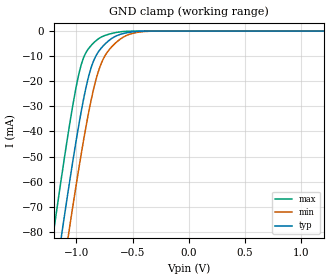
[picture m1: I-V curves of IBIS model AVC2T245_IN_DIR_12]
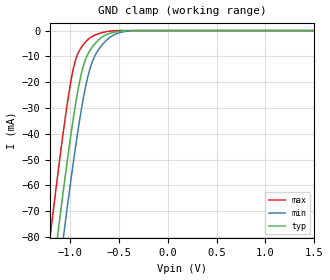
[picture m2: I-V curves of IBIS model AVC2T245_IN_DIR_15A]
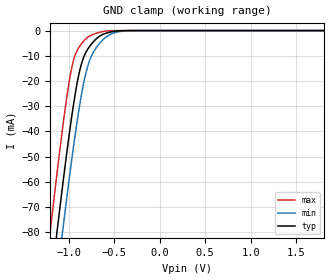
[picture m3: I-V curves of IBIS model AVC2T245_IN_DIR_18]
| TEXAS INSTRUMENTS INCORPORATED
| Standard Linear and Logic Group
| IBIS Model of SN74AVC2T245
| Dual-Bit Dual-Supply Bus Transceiver With Configurable Voltage
| Translation and 3-State Outputs
| This file contains package information for the following:
|  LGA 10-pin (RSW) package as [Component] SN74AVC2T245_RSW
| This device can be powered at the following Vccs:
|  1.2 volt Vcc
|  1.5 volt Vcc
|  1.8 volt Vcc
|  2.5 volt Vcc
|  3.3 volt Vcc
| This file provides unique models under the [Model Selector] for each Vcc.
| For operation at a specific Vcc, select the appropriate model after each
| [Model Selector] keyword.
[IBIS Ver]   3.2
[Comment char]  |_char
[File Name]   sn74avc2t245.ibs
[File Rev]   1.1 | x_die
[Date]   January 7, 2009
[Source]   Data created from TI-SPICE simulations at TI-SLL.
[Notes]   The following is an IBIS list for the SN74AVC2T245.
   Please contact sllibis@ti.com with questions and
   comments concerning SLL IBIS models.
   -FILE REV HISTORY
   -1.1 Release IBIS file on 01/08/09.
   -Power Clamp data deleted from control input model as there
   is no power-clamp diode.
[Disclaimer] Property of Texas Instruments Incorporated.  Unauthorized
   reproduction and/or distribution is strictly prohibited.
   This product is protected under copyright law.
   Created  2009, (C) Copyright  2009, Texas Instruments
   Incorporated, All Rights Reserved
   UNLESS THERE IS A SIGNED, WRITTEN AGREEMENT TO THE
   CONTRARY, TEXAS INSTRUMENTS (TI) IS PROVIDING THE IBIS
   MODELS  AND WITHOUT ANY WARRANTY, EXPRESSED OR
   IMPLIED.  TI assumes no liability for:
   1) the accuracy of the IBIS models provided to your
   company;
   2) the proper functioning of these IBIS Models in your
   design or for any resulting applications; or
   3) infringement of patents, copyrights or intellectual
   property rights resulting from your use of these IBIS
   models.
   TI provides IBIS Models as a service to our customers.
   You and your company shall not distribute, sell or give
   these models to anyone else without prior written
   permission from TI.
   TI reserves the right to make changes to our products or
   to discontinue any semiconductor product or service
   without notice, and advises our customers to obtain the
   latest version of relevant information to verify, before
   placing orders, that the information being relied on is
   current.
   Please be aware that your receipt and use of the IBIS
   information provided shall serve as acceptance of these
   terms and conditions.  If you do not accept these terms,
   you should return or destroy the IBIS models and any
   other accompanying information immediately.
| Component SN74AVC2T245_RSW 10-PIN LGA
[Component]   SN74AVC2T245_RSW
[Manufacturer]   Texas Instruments, Inc.
[Package]
|   typ   min   max
R_pkg   1.700e-02   1.500e-02   2.200e-02
L_pkg   5.570e-10   4.830e-10   6.520e-10
C_pkg   1.440e-13   1.050e-13   1.870e-13
[Pin]   signal_name   model_name   R_pin   L_pin   C_pin
1   DIR2   AVC2T245_IN_DIR   1.600e-02   4.830e-10   1.100e-13
2   NOE   AVC2T245_IN_NOE   1.500e-02   5.130e-10   1.860e-13
3   GND   GND   1.800e-02   5.860e-10   1.870e-13
4   B2   AVC2T245_IO   2.200e-02   6.520e-10   1.180e-13
5   B1   AVC2T245_IO   1.600e-02   5.500e-10   1.250e-13
6   VCCB   POWER   1.600e-02   4.830e-10   1.050e-13
7   VCCA   POWER   1.500e-02   5.150e-10   1.820e-13
8   A1   AVC2T245_IO   1.700e-02   5.790e-10   1.870e-13
9   A2   AVC2T245_IO   2.200e-02   6.360e-10   1.170e-13
10   DIR1   AVC2T245_IN_DIR   1.700e-02   5.710e-10   1.280e-13
| Model AVC2T245_IN_DIR
[Model Selector]   AVC2T245_IN_DIR
AVC2T245_IN_DIR_12   1.2 volt Vcc
AVC2T245_IN_DIR_15A   1.5 volt Vcc
AVC2T245_IN_DIR_18   1.8 volt Vcc
AVC2T245_IN_DIR_25   2.5 volt Vcc
AVC2T245_IN_DIR_33   3.3 volt Vcc
| Model AVC2T245_IN_NOE
[Model Selector]   AVC2T245_IN_NOE
AVC2T245_IN_NOE_12   1.2 volt Vcc
AVC2T245_IN_NOE_15A   1.5 volt Vcc
AVC2T245_IN_NOE_18   1.8 volt Vcc
AVC2T245_IN_NOE_25   2.5 volt Vcc
AVC2T245_IN_NOE_33   3.3 volt Vcc
| Model AVC2T245_IO
[Model Selector]   AVC2T245_IO
AVC2T245_IO_12   1.2 volt Vcc
AVC2T245_IO_15A   1.5 volt Vcc
AVC2T245_IO_18   1.8 volt Vcc
AVC2T245_IO_25   2.5 volt Vcc
AVC2T245_IO_33   3.3 volt Vcc
| Models and submodels in the file (15): AVC2T245_IN_DIR_12 (Input), AVC2T245_IN_DIR_15A (Input), AVC2T245_IN_DIR_18 (Input), AVC2T245_IN_DIR_25 (Input), AVC2T245_IN_DIR_33 (Input), AVC2T245_IN_NOE_12 (Input), AVC2T245_IN_NOE_15A (Input), AVC2T245_IN_NOE_18 (Input), AVC2T245_IN_NOE_25 (Input), AVC2T245_IN_NOE_33 (Input), AVC2T245_IO_12 (I/O), AVC2T245_IO_15A (I/O), AVC2T245_IO_18 (I/O), AVC2T245_IO_25 (I/O), AVC2T245_IO_33 (I/O)
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[Model]   AVC2T245_IN_DIR_12
Model_type  Input
Vinl=0.385
Vinh=0.845
| variable   typ   min   max
C_comp   2.12pF   1.85pF   2.57pF
[Temperature Range]   40   100   -40
| Ambient temperature   25   85   -40
[Voltage range]   1.2   1.1   1.3
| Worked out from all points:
|   GND clamp passes 1 mA (typ) near -0.58 V on its own axis
[GND Clamp]
| AVC2T245_IN_DIR_12
|   Voltage   I(typ)   I(min)   I(max)
-4.6V     -1.266A    -1.277A    -1.254A
-1.22V    -108.9mA   -127.3mA   -85.71mA
-1.195V   -101.1mA   -119.4mA   -77.82mA
-1.13V    -81mA      -99.35mA   -57.75mA
-1.065V   -61.6mA    -79.78mA   -38.73mA
-960mV    -32.94mA   -49.96mA   -14.03mA
-905mV    -20.72mA   -35.89mA   -7.898mA
-860mV    -13.49mA   -25.81mA   -5.335mA
-760mV    -5.854mA   -11.09mA   -2.009mA
-615mV    -1.4mA     -3.395mA   -339.9uA
-340mV    -6.933uA   -59.17uA   -50.62nA
1.2V      105.6pA    10.37nA    15.63pA
[Model]   AVC2T245_IN_DIR_15A
Model_type  Input
Vinl=0.49
Vinh=1.04
| variable   typ   min   max
C_comp   2.08pF   1.77pF   2.54pF
[Temperature Range]   40   100   -40
| Ambient temperature   25   85   -40
[Voltage range]   1.5   1.4   1.6
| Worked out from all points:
|   GND clamp passes 1 mA (typ) near -0.58 V on its own axis
[GND Clamp]
| AVC2T245_IN_DIR_15A
|   Voltage   I(typ)   I(min)   I(max)
-4.6V     -1.266A    -1.277A    -1.254A
-1.21V    -105.8mA   -124.1mA   -82.55mA
-1.185V   -97.95mA   -116.3mA   -74.69mA
-1.125V   -79.48mA   -97.82mA   -56.25mA
-1.06V    -60.14mA   -78.3mA    -37.34mA
-960mV    -32.94mA   -49.96mA   -14.03mA
-865mV    -14.14mA   -26.84mA   -5.576mA
-810mV    -8.703mA   -16.94mA   -3.298mA
-765mV    -6.095mA   -11.55mA   -2.106mA
-600mV    -1.191mA   -2.914mA   -255.1uA
-325mV    -4.51uA    -42.57uA   -26.57nA
1.5V      116.5pA    11.58nA    19.54pA
[Model]   AVC2T245_IN_DIR_18
Model_type  Input
Vinl=0.5775
Vinh=1.2675
| variable   typ   min   max
C_comp   2.04pF   1.70pF   2.53pF
[Temperature Range]   40   100   -40
| Ambient temperature   25   85   -40
[Voltage range]   1.8   1.65   1.95
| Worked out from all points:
|   GND clamp passes 1 mA (typ) near -0.58 V on its own axis
[GND Clamp]
| AVC2T245_IN_DIR_18
|   Voltage   I(typ)   I(min)   I(max)
-4.6V     -1.266A    -1.277A    -1.254A
-1.2V     -102.6mA   -121mA     -79.39mA
-1.135V   -82.53mA   -100.9mA   -59.27mA
-1.115V   -76.45mA   -94.78mA   -53.25mA
-1.065V   -61.6mA    -79.78mA   -38.73mA
-960mV    -32.94mA   -49.96mA   -14.03mA
-905mV    -20.72mA   -35.89mA   -7.898mA
-860mV    -13.49mA   -25.81mA   -5.335mA
-760mV    -5.854mA   -11.09mA   -2.009mA
-585mV    -1.007mA   -2.481mA   -186.3uA
-310mV    -2.903uA   -30.35uA   -13.82nA
1.8V      127.8pA    12.94nA    23.41pA
